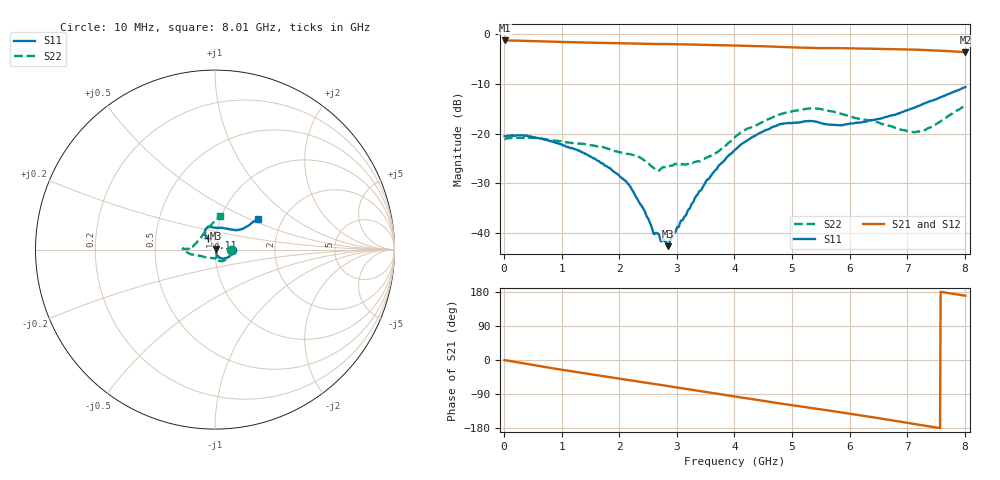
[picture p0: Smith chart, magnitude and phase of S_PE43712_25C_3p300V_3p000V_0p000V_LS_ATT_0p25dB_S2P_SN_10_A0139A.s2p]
! DEVICE ID: PE43712
! File Path: z:\PE43713\PE43713_CHAR_NOM_04292014\AMB\3p300\LS_ATT_0p25dB\PE43713_AMB_3p300V_3p000V_0p000V_LS_ATT_0p25dB_S2P_SN_10_A0139A.s2p
! Serial: 10
! Lot: A0139A
! Temp: 25C
! VDD: 3.300
! VSS: 0.000
! Control_Hi: 3.000
! Control_Lo: 0.000
! Attenuation Step: 0.25dB
! Port 1: RF1
! Port 2: RF2
! ThroughPath:1-2
! IDD: 0.0001468006
! ISS: -3.74e-008
#  Hz  S  RI  R  50
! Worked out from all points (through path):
!   801 points, 10 MHz to 8.01 GHz, reference 50 ohm
!   highest |S21| = -1.22 dB at 10 MHz (marker M1); lowest = -3.6 dB at 8.01 GHz (marker M2)
!   group delay of S21, straight-line fit = 65.1 ps
!   lowest |S11| = -42.7 dB at 2.85 GHz (marker M3), VSWR 1.01, Z = 50.5 + j0.501 ohm
!   |S11| at or under -10 dB: start of sweep to end of sweep
!   |S22| runs from -27.6 to -14.4 dB; largest |S21 - S12| = 0.003
!   S11 on the Smith chart (normalised r, x): 10 MHz: 1.21, -0.00; 4.11 GHz: 0.91, +0.12; 8.01 GHz: 1.50, +0.56
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1e7  0.0939 -0.000615  0.8688 -0.00487  0.8685 -0.00462  0.0883 -0.000953
3.6e8  0.0922 -0.0239  0.8483 -0.1432  0.8505 -0.1427  0.0862 -0.0244
6.9e8  0.0782 -0.0386  0.8091 -0.2634  0.8085 -0.2632  0.0774 -0.041
1.35e9  0.0409 -0.0501  0.6882 -0.4632  0.6878 -0.4629  0.0471 -0.0629
1.82e9  0.0203 -0.0404  0.5793 -0.5773  0.5789 -0.577  0.0279 -0.0637
2.14e9  0.00935 -0.0302  0.4951 -0.6429  0.4949 -0.6425  0.0138 -0.0607
2.42e9  0.008 -0.0155  0.4152 -0.6902  0.4153 -0.6898  0.0105 -0.0532
2.59e9  0.00849 -0.00529  0.3652 -0.7123  0.3652 -0.7124  0.00802 -0.0446
2.68e9  0.0097 -8.75e-05  0.3396 -0.7237  0.3398 -0.7232  0.011 -0.0405
2.75e9  0.00831 0.00125  0.3193 -0.7334  0.3194 -0.733  0.0102 -0.0441
2.85e9  0.00536 0.00496  0.2873 -0.7443  0.2875 -0.7444  0.00344 -0.0468
3.43e9  -0.0096 0.0256  0.1009 -0.779  0.1012 -0.7793  -0.0272 -0.0461
3.74e9  -0.0198 0.044  0.00188 -0.7806  0.00273 -0.7805  -0.0523 -0.0424
4.01e9  -0.035 0.0587  -0.0855 -0.7687  -0.0848 -0.7684  -0.0852 -0.0352
4.11e9  -0.0415 0.0653  -0.1165 -0.76  -0.1164 -0.7602  -0.0972 -0.0331
4.78e9  -0.0538 0.1115  -0.3082 -0.6817  -0.3075 -0.6822  -0.1544 -0.0158
5.35e9  -0.0324 0.1295  -0.44 -0.5838  -0.4398 -0.583  -0.18 0.00433
5.85e9  0.0113 0.1205  -0.5422 -0.4836  -0.5409 -0.4839  -0.1581 0.00398
6.68e9  0.1007 0.1106  -0.6585 -0.2676  -0.6583 -0.267  -0.1176 0.0222
7.05e9  0.1369 0.1111  -0.6859 -0.1586  -0.6852 -0.1586  -0.0878 0.0554
7.26e9  0.1586 0.117  -0.6906 -0.0946  -0.6898 -0.0943  -0.0662 0.0828
8.01e9  0.2387 0.1705  -0.6518 0.1181  -0.6496 0.1168  0.0255 0.1893
